(* Logix 5000 Program export KEP; software revision 30.00; part 6 of 15 *)

ADD_ON_INSTRUCTION L_INC   (* revision 1.0 00 Release, vendor Rockwell Automation *)
// Increment (64-bit)
// Revision note:
// Initial Release
// Help:
// This instruction increments the input 64-bit integer, returning its value plus 1.
VAR_IN_OUT
   Inp : LINT; {required}   // Input
   Out : LINT; {required}   // Output = Input + 1
END_VAR
VAR
   Wrk : DINT[2];   // Working pair of 32-bit integers (DINTs)
   Wrk_LoOvflw : BOOL;   // Low-order 32-bit overflow (without minor fault)
   Wrk_HiOvflw : BOOL;   // High-order 32-bit overflow (without minor fault)
END_VAR

ROUTINE Logic   (* ladder *)
// Output the value of the input plus 1
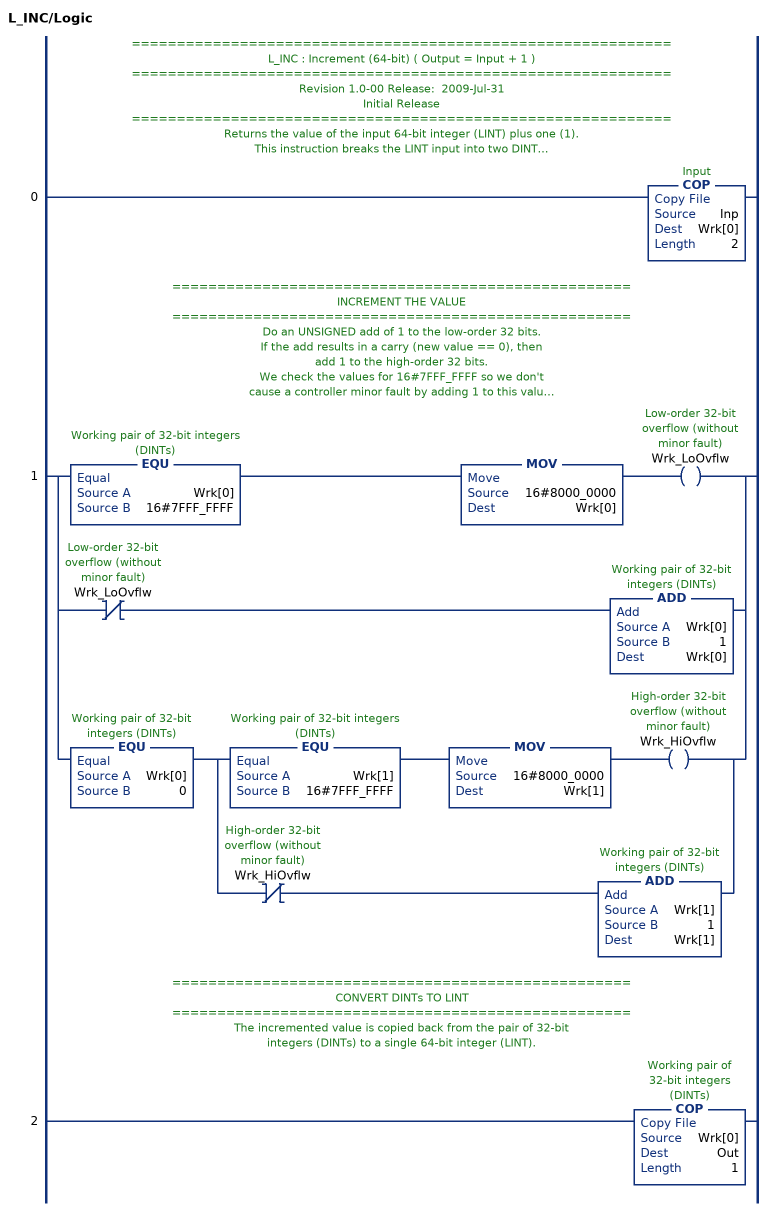
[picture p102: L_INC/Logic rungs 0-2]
   // ============================================================
   // L_INC : Increment (64-bit) ( Output = Input + 1 )
   // ============================================================
   // Revision 1.0-00 Release:  2009-Jul-31
   // Initial Release
   // ============================================================
   // Returns the value of the input 64-bit integer (LINT) plus one (1).
   // This instruction breaks the LINT input into two DINTs
   // (32-bit signed each) to do the math.
   // ===================================================
   // CONVERT LINT TO DINTs
   // ===================================================
   // This COPy takes the input LINT and breaks it into a pair of DINTs.
   0: COP(Inp,Wrk[0],2);
   // ===================================================
   // INCREMENT THE VALUE
   // ===================================================
   // Do an UNSIGNED add of 1 to the low-order 32 bits.
   // If the add results in a carry (new value == 0), then
   // add 1 to the high-order 32 bits.
   // We check the values for 16#7FFF_FFFF so we don't
   // cause a controller minor fault by adding 1 to this value
   // (resulting in a signed overflow to negative).
   1: [EQU(Wrk[0],16#7FFF_FFFF) MOV(16#8000_0000,Wrk[0]) OTE(Wrk_LoOvflw) ,XIO(Wrk_LoOvflw) ADD(Wrk[0],1,Wrk[0]) ,EQU(Wrk[0],0) [EQU(Wrk[1],16#7FFF_FFFF) MOV(16#8000_0000,Wrk[1]) OTE(Wrk_HiOvflw) ,XIO(Wrk_HiOvflw) ADD(Wrk[1],1,Wrk[1]) ] ];
   // ===================================================
   // CONVERT DINTs TO LINT
   // ===================================================
   // The incremented value is copied back from the pair of 32-bit
   // integers (DINTs) to a single 64-bit integer (LINT).
   2: COP(Wrk[0],Out,1);
END_ROUTINE
END_ADD_ON_INSTRUCTION

ADD_ON_INSTRUCTION Ed25519_SIGN   (* revision 1.0 20170916, vendor Kenneth A. Fischer *)
// Generates an Ed25519 Signature.
// Revision note:
// Rev1.0: 20170916 - Initial Release
VAR_IN_OUT
   Temp_C1 : DINT[22]; {required}   // Temp C1 value
   Temp_C2 : DINT[22]; {required}   // Temp C2 value
   Temp_C3 : DINT[22]; {required}   // Temp C3 value
   Temp_C4 : DINT[22]; {required}   // Temp C4 value
   Temp_C5 : DINT[22]; {required}   // Temp C5 value
   Temp_C6 : DINT[22]; {required}   // Temp C6 value
   Temp_C7 : DINT[22]; {required}   // Temp C7 value
   Temp_C8 : DINT[22]; {required}   // Temp C8 value
   Temp_C9 : DINT[22]; {required}   // Temp C9 value
   Temp_C10 : DINT[22]; {required}   // Temp C10 value
   Temp_D1 : DINT[43]; {required}   // Temp D1 Value, w at steps 4/5 and 13/14
   Temp_D2 : DINT[43]; {required}
   Temp_E1 : DINT[32]; {required}   // Temp E1 Value, re
   Temp_E2 : DINT[32]; {required}   // Temp E2 Value, SIG_R between steps 8 and 9, ke for rest
   Temp_E3 : DINT[32]; {required}
   Temp_L : LINT[4]; {required}   // Temp L value
   Temp_S : STRING; {required}   // Temp String
   Temp_P1 : POINT; {required}   // Base Point B
   Temp_P2 : POINT; {required}   // Temp Point for Multiplication
   Temp_P3 : POINT; {required}   // Signature R as Point before encoding
   Temp_P4 : POINT; {required}
   Temp_MSG : LINT[1600]; {required}
   Temp_HASH : LINT[8]; {required}
   Inp_Flags : DINT; {required}
   Inp_PubDH : STRING; {required}
   Inp_Ke : STRING; {required}
   Inp_KsID : LINT; {required}
   Inp_KsPrimeID : LINT; {required}
   Inp_PubKey : STRING; {required}
   Inp_PriKey_scalar : STRING; {required}
   Inp_PriKey_prefix : STRING; {required}
   Out_Counter : LINT; {required}
   Out_Sig_R : STRING; {required}
   Out_Sig_S : STRING; {required}
END_VAR
VAR_OUTPUT
   SEQCTRL_DN : BOOL; {access Read Only}   // Complete
END_VAR
VAR_INPUT
   SEQCTRL_RESET : BOOL;   // Resets Ed25519 Sign if Toggled True
END_VAR
VAR_OUTPUT
   SEQCTRL_STEP : INT; {access Read Only}
   SEQCTRL_SUBSTEP : INT; {access Read Only}
END_VAR
VAR
   SEQCTRL_CMD : DINT;
   SEQCTRL_CMD_TABLE : DINT[70];
   SEQCTRL_DONE : DINT;
   SEQCTRL_NEXT_STEP : INT;
   i : INT;
   TEMP : DINT;
   SHA512_SEQ1 : SHA512_SEQ;
   SEQCTRL_ONS : DINT;
   B512_HtoD : B512_HtoD;
   B256_MODL1 : B256_MODL;
   POINT_MUL : POINT_MUL;
   POINT_ENC : POINT_ENC;
   B256_EtoC : B256_EtoC;
   B256_CtoS : B256_CtoS;
   SHA512_SEQ2 : SHA512_SEQ;
   B256_MODL2 : B256_MODL;
   j : INT;
   B256_NNRED : B256_NNRED;
   B256_EtoL : B256_EtoL;
   B256_StoC : B256_StoC;
   B256_CtoE : B256_CtoE;
   B256_StoSLE : B256_StoSLE;
   Wrk_Out : DINT[2];
   L_INC : L_INC;
END_VAR

ROUTINE Logic   (* ladder *)
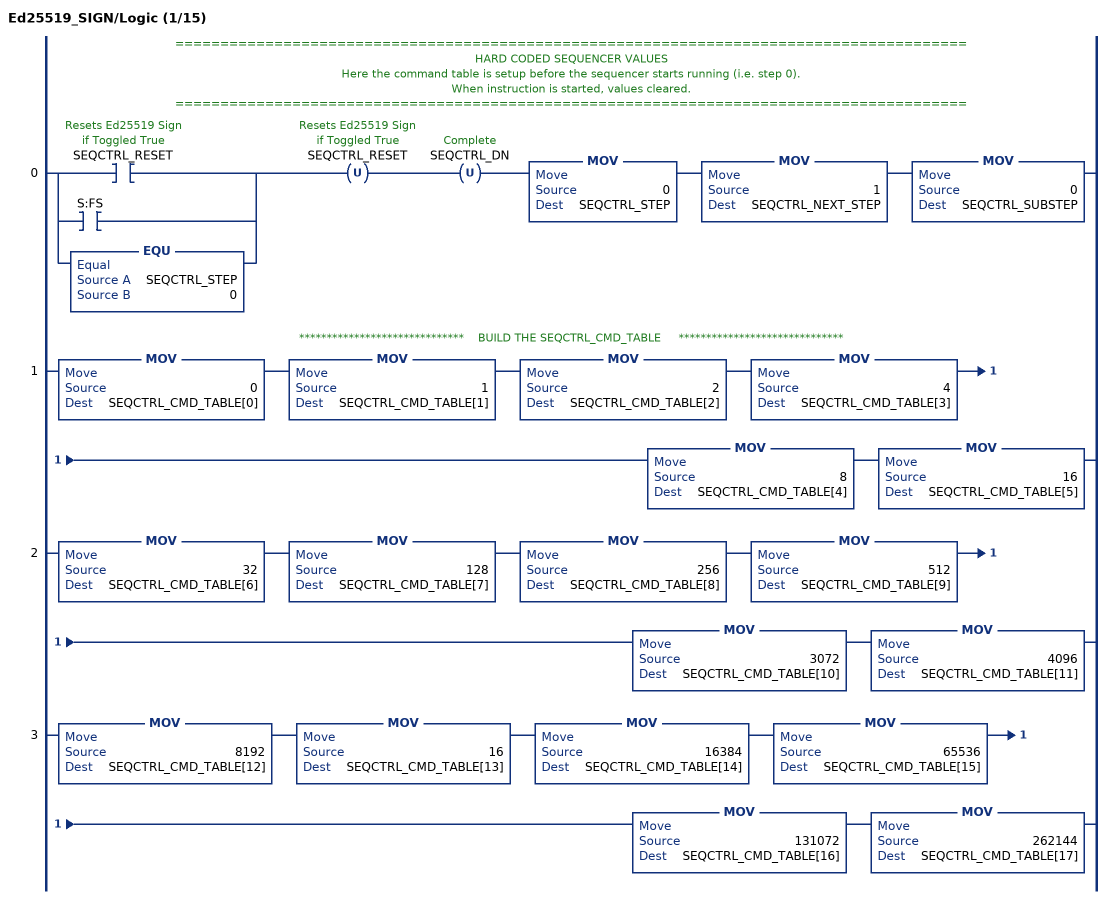
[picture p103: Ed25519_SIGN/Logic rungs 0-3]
   // ========================================================================================
   // HARD CODED SEQUENCER VALUES
   // Here the command table is setup before the sequencer starts running (i.e. step 0).
   // When instruction is started, values cleared.
   // ========================================================================================
   0: [[XIC(SEQCTRL_RESET) ,XIC(S:FS) ] ,EQU(SEQCTRL_STEP,0) ]OTU(SEQCTRL_RESET)OTU(SEQCTRL_DN)MOV(0,SEQCTRL_STEP)MOV(1,SEQCTRL_NEXT_STEP)MOV(0,SEQCTRL_SUBSTEP);
   // ******************************    BUILD THE SEQCTRL_CMD_TABLE     ******************************
   1: MOV(0,SEQCTRL_CMD_TABLE[0])MOV(1,SEQCTRL_CMD_TABLE[1])MOV(2,SEQCTRL_CMD_TABLE[2])MOV(4,SEQCTRL_CMD_TABLE[3])MOV(8,SEQCTRL_CMD_TABLE[4])MOV(16,SEQCTRL_CMD_TABLE[5]);
   2: MOV(32,SEQCTRL_CMD_TABLE[6])MOV(128,SEQCTRL_CMD_TABLE[7])MOV(256,SEQCTRL_CMD_TABLE[8])MOV(512,SEQCTRL_CMD_TABLE[9])MOV(3072,SEQCTRL_CMD_TABLE[10])MOV(4096,SEQCTRL_CMD_TABLE[11]);
   3: MOV(8192,SEQCTRL_CMD_TABLE[12])MOV(16,SEQCTRL_CMD_TABLE[13])MOV(16384,SEQCTRL_CMD_TABLE[14])MOV(65536,SEQCTRL_CMD_TABLE[15])MOV(131072,SEQCTRL_CMD_TABLE[16])MOV(262144,SEQCTRL_CMD_TABLE[17]);
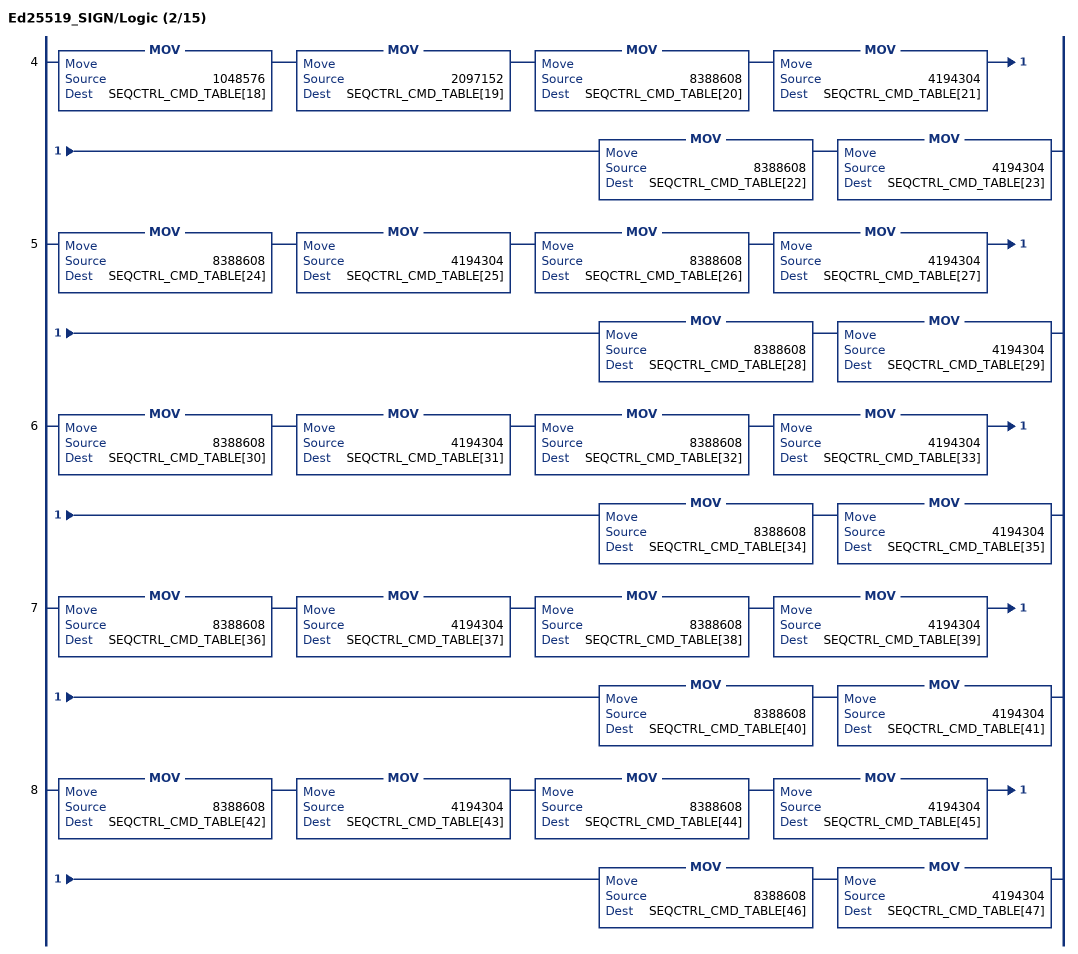
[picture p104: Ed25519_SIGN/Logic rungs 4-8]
   4: MOV(1048576,SEQCTRL_CMD_TABLE[18])MOV(2097152,SEQCTRL_CMD_TABLE[19])MOV(8388608,SEQCTRL_CMD_TABLE[20])MOV(4194304,SEQCTRL_CMD_TABLE[21])MOV(8388608,SEQCTRL_CMD_TABLE[22])MOV(4194304,SEQCTRL_CMD_TABLE[23]);
   5: MOV(8388608,SEQCTRL_CMD_TABLE[24])MOV(4194304,SEQCTRL_CMD_TABLE[25])MOV(8388608,SEQCTRL_CMD_TABLE[26])MOV(4194304,SEQCTRL_CMD_TABLE[27])MOV(8388608,SEQCTRL_CMD_TABLE[28])MOV(4194304,SEQCTRL_CMD_TABLE[29]);
   6: MOV(8388608,SEQCTRL_CMD_TABLE[30])MOV(4194304,SEQCTRL_CMD_TABLE[31])MOV(8388608,SEQCTRL_CMD_TABLE[32])MOV(4194304,SEQCTRL_CMD_TABLE[33])MOV(8388608,SEQCTRL_CMD_TABLE[34])MOV(4194304,SEQCTRL_CMD_TABLE[35]);
   7: MOV(8388608,SEQCTRL_CMD_TABLE[36])MOV(4194304,SEQCTRL_CMD_TABLE[37])MOV(8388608,SEQCTRL_CMD_TABLE[38])MOV(4194304,SEQCTRL_CMD_TABLE[39])MOV(8388608,SEQCTRL_CMD_TABLE[40])MOV(4194304,SEQCTRL_CMD_TABLE[41]);
   8: MOV(8388608,SEQCTRL_CMD_TABLE[42])MOV(4194304,SEQCTRL_CMD_TABLE[43])MOV(8388608,SEQCTRL_CMD_TABLE[44])MOV(4194304,SEQCTRL_CMD_TABLE[45])MOV(8388608,SEQCTRL_CMD_TABLE[46])MOV(4194304,SEQCTRL_CMD_TABLE[47]);
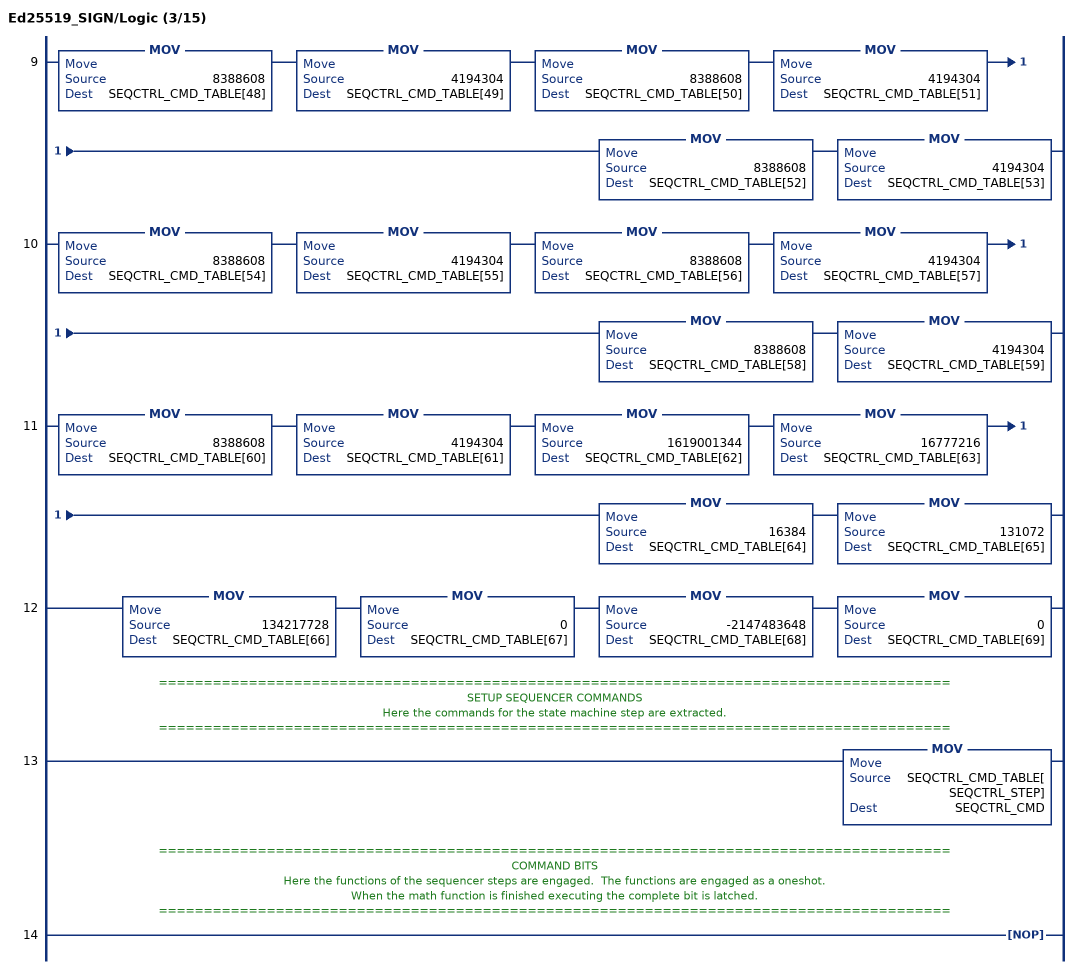
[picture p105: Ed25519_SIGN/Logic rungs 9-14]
   9: MOV(8388608,SEQCTRL_CMD_TABLE[48])MOV(4194304,SEQCTRL_CMD_TABLE[49])MOV(8388608,SEQCTRL_CMD_TABLE[50])MOV(4194304,SEQCTRL_CMD_TABLE[51])MOV(8388608,SEQCTRL_CMD_TABLE[52])MOV(4194304,SEQCTRL_CMD_TABLE[53]);
   10: MOV(8388608,SEQCTRL_CMD_TABLE[54])MOV(4194304,SEQCTRL_CMD_TABLE[55])MOV(8388608,SEQCTRL_CMD_TABLE[56])MOV(4194304,SEQCTRL_CMD_TABLE[57])MOV(8388608,SEQCTRL_CMD_TABLE[58])MOV(4194304,SEQCTRL_CMD_TABLE[59]);
   11: MOV(8388608,SEQCTRL_CMD_TABLE[60])MOV(4194304,SEQCTRL_CMD_TABLE[61])MOV(1619001344,SEQCTRL_CMD_TABLE[62])MOV(16777216,SEQCTRL_CMD_TABLE[63])MOV(16384,SEQCTRL_CMD_TABLE[64])MOV(131072,SEQCTRL_CMD_TABLE[65]);
   12: MOV(134217728,SEQCTRL_CMD_TABLE[66])MOV(0,SEQCTRL_CMD_TABLE[67])MOV(-2147483648,SEQCTRL_CMD_TABLE[68])MOV(0,SEQCTRL_CMD_TABLE[69]);
   // ========================================================================================
   // SETUP SEQUENCER COMMANDS
   // Here the commands for the state machine step are extracted.
   // ========================================================================================
   13: MOV(SEQCTRL_CMD_TABLE[SEQCTRL_STEP],SEQCTRL_CMD);
   // ========================================================================================
   // COMMAND BITS
   // Here the functions of the sequencer steps are engaged.  The functions are engaged as a oneshot.
   // When the math function is finished executing the complete bit is latched.
   // ========================================================================================
   14: NOP();
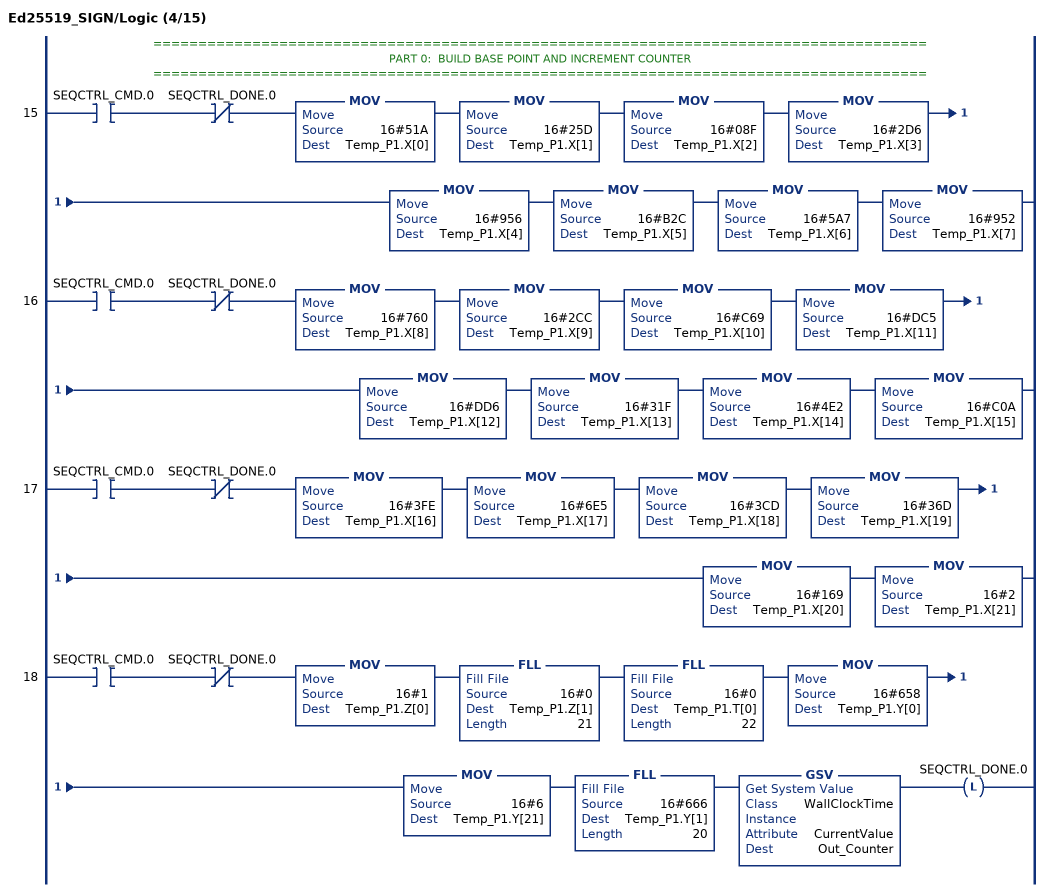
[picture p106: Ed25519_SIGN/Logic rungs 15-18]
   // ======================================================================================
   // PART 0:  BUILD BASE POINT AND INCREMENT COUNTER
   // ======================================================================================
   15: XIC(SEQCTRL_CMD.0)XIO(SEQCTRL_DONE.0)MOV(16#51A,Temp_P1.X[0])MOV(16#25D,Temp_P1.X[1])MOV(16#08F,Temp_P1.X[2])MOV(16#2D6,Temp_P1.X[3])MOV(16#956,Temp_P1.X[4])MOV(16#B2C,Temp_P1.X[5])MOV(16#5A7,Temp_P1.X[6])MOV(16#952,Temp_P1.X[7]);
   16: XIC(SEQCTRL_CMD.0)XIO(SEQCTRL_DONE.0)MOV(16#760,Temp_P1.X[8])MOV(16#2CC,Temp_P1.X[9])MOV(16#C69,Temp_P1.X[10])MOV(16#DC5,Temp_P1.X[11])MOV(16#DD6,Temp_P1.X[12])MOV(16#31F,Temp_P1.X[13])MOV(16#4E2,Temp_P1.X[14])MOV(16#C0A,Temp_P1.X[15]);
   17: XIC(SEQCTRL_CMD.0)XIO(SEQCTRL_DONE.0)MOV(16#3FE,Temp_P1.X[16])MOV(16#6E5,Temp_P1.X[17])MOV(16#3CD,Temp_P1.X[18])MOV(16#36D,Temp_P1.X[19])MOV(16#169,Temp_P1.X[20])MOV(16#2,Temp_P1.X[21]);
   18: XIC(SEQCTRL_CMD.0)XIO(SEQCTRL_DONE.0)MOV(16#1,Temp_P1.Z[0])FLL(16#0,Temp_P1.Z[1],21)FLL(16#0,Temp_P1.T[0],22)MOV(16#658,Temp_P1.Y[0])MOV(16#6,Temp_P1.Y[21])FLL(16#666,Temp_P1.Y[1],20)GSV(WallClockTime,,CurrentValue,Out_Counter)OTL(SEQCTRL_DONE.0);
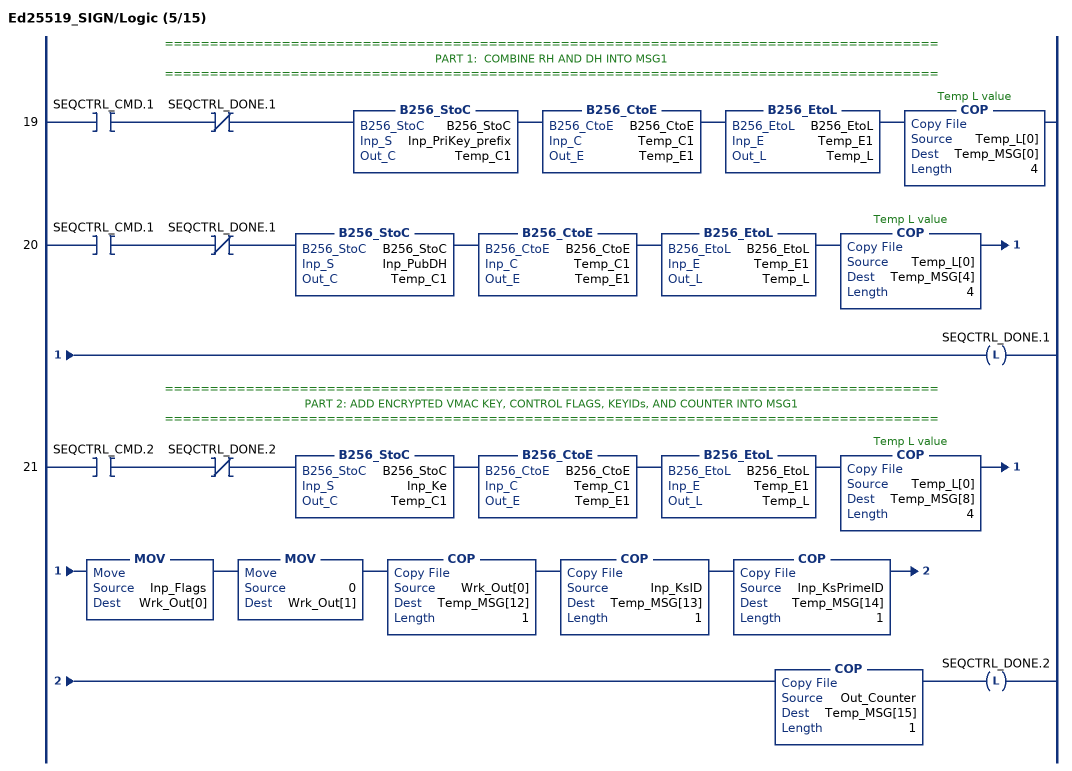
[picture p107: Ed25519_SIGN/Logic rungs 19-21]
   // ======================================================================================
   // PART 1:  COMBINE RH AND DH INTO MSG1
   // ======================================================================================
   19: XIC(SEQCTRL_CMD.1)XIO(SEQCTRL_DONE.1)B256_StoC(B256_StoC,Inp_PriKey_prefix,Temp_C1)B256_CtoE(B256_CtoE,Temp_C1,Temp_E1)B256_EtoL(B256_EtoL,Temp_E1,Temp_L)COP(Temp_L[0],Temp_MSG[0],4);
   20: XIC(SEQCTRL_CMD.1)XIO(SEQCTRL_DONE.1)B256_StoC(B256_StoC,Inp_PubDH,Temp_C1)B256_CtoE(B256_CtoE,Temp_C1,Temp_E1)B256_EtoL(B256_EtoL,Temp_E1,Temp_L)COP(Temp_L[0],Temp_MSG[4],4)OTL(SEQCTRL_DONE.1);
   // ======================================================================================
   // PART 2: ADD ENCRYPTED VMAC KEY, CONTROL FLAGS, KEYIDs, AND COUNTER INTO MSG1
   // ======================================================================================
   21: XIC(SEQCTRL_CMD.2)XIO(SEQCTRL_DONE.2)B256_StoC(B256_StoC,Inp_Ke,Temp_C1)B256_CtoE(B256_CtoE,Temp_C1,Temp_E1)B256_EtoL(B256_EtoL,Temp_E1,Temp_L)COP(Temp_L[0],Temp_MSG[8],4)MOV(Inp_Flags,Wrk_Out[0])MOV(0,Wrk_Out[1])COP(Wrk_Out[0],Temp_MSG[12],1)COP(Inp_KsID,Temp_MSG[13],1)COP(Inp_KsPrimeID,Temp_MSG[14],1)COP(Out_Counter,Temp_MSG[15],1)OTL(SEQCTRL_DONE.2);
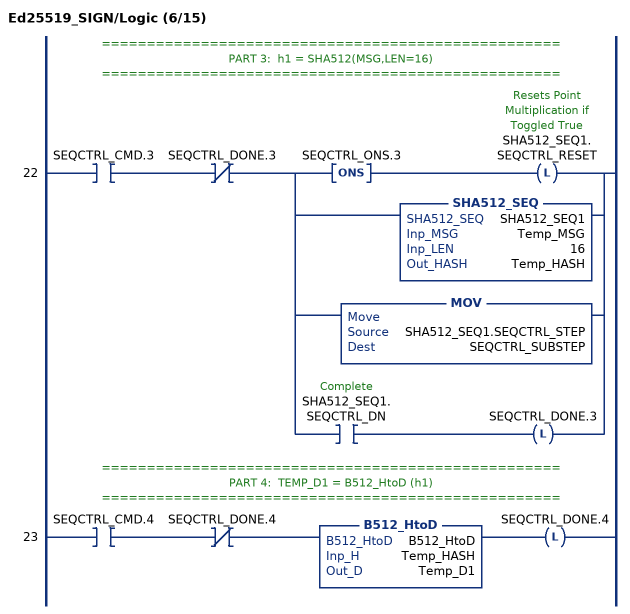
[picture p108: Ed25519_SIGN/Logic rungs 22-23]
   // ===================================================
   // PART 3:  h1 = SHA512(MSG,LEN=16)
   // ===================================================
   22: XIC(SEQCTRL_CMD.3)XIO(SEQCTRL_DONE.3)[ONS(SEQCTRL_ONS.3) OTL(SHA512_SEQ1.SEQCTRL_RESET) ,SHA512_SEQ(SHA512_SEQ1,Temp_MSG,16,Temp_HASH) ,MOV(SHA512_SEQ1.SEQCTRL_STEP,SEQCTRL_SUBSTEP) ,XIC(SHA512_SEQ1.SEQCTRL_DN) OTL(SEQCTRL_DONE.3) ];
   // ===================================================
   // PART 4:  TEMP_D1 = B512_HtoD (h1)
   // ===================================================
   23: XIC(SEQCTRL_CMD.4)XIO(SEQCTRL_DONE.4)B512_HtoD(B512_HtoD,Temp_HASH,Temp_D1)OTL(SEQCTRL_DONE.4);
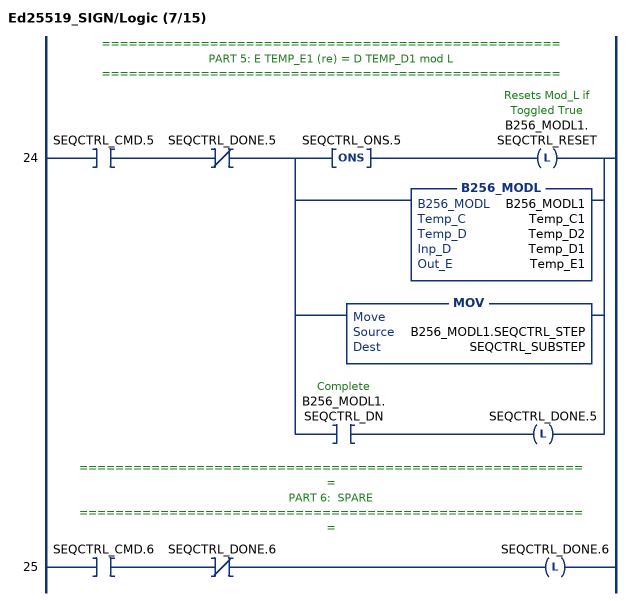
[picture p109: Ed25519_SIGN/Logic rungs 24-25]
   // ===================================================
   // PART 5: E TEMP_E1 (re) = D TEMP_D1 mod L
   // ===================================================
   24: XIC(SEQCTRL_CMD.5)XIO(SEQCTRL_DONE.5)[ONS(SEQCTRL_ONS.5) OTL(B256_MODL1.SEQCTRL_RESET) ,B256_MODL(B256_MODL1,Temp_C1,Temp_D2,Temp_D1,Temp_E1) ,MOV(B256_MODL1.SEQCTRL_STEP,SEQCTRL_SUBSTEP) ,XIC(B256_MODL1.SEQCTRL_DN) OTL(SEQCTRL_DONE.5) ];
   // =========================================================
   // PART 6:  SPARE
   // =========================================================
   25: XIC(SEQCTRL_CMD.6)XIO(SEQCTRL_DONE.6)OTL(SEQCTRL_DONE.6);
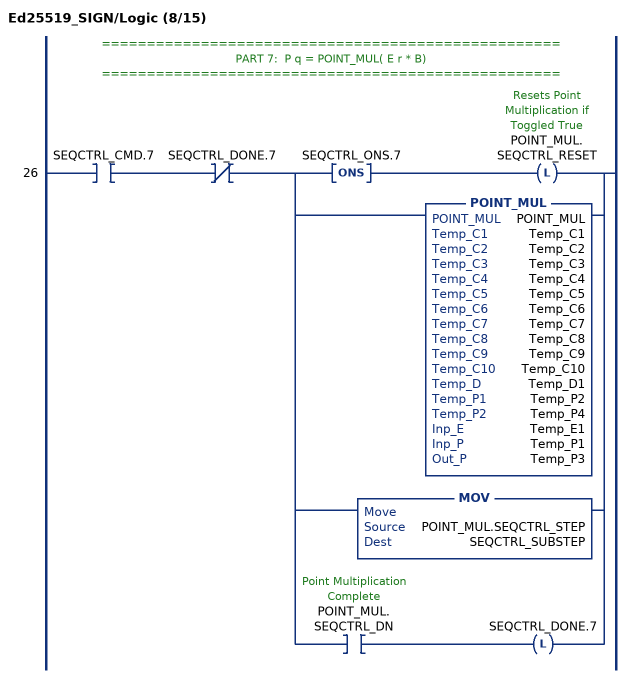
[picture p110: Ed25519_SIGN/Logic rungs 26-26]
   // ===================================================
   // PART 7:  P q = POINT_MUL( E r * B)
   // ===================================================
   26: XIC(SEQCTRL_CMD.7)XIO(SEQCTRL_DONE.7)[ONS(SEQCTRL_ONS.7) OTL(POINT_MUL.SEQCTRL_RESET) ,POINT_MUL(POINT_MUL,Temp_C1,Temp_C2,Temp_C3,Temp_C4,Temp_C5,Temp_C6,Temp_C7,Temp_C8,Temp_C9,Temp_C10,Temp_D1,Temp_P2,Temp_P4,Temp_E1,Temp_P1,Temp_P3) ,MOV(POINT_MUL.SEQCTRL_STEP,SEQCTRL_SUBSTEP) ,XIC(POINT_MUL.SEQCTRL_DN) OTL(SEQCTRL_DONE.7) ];
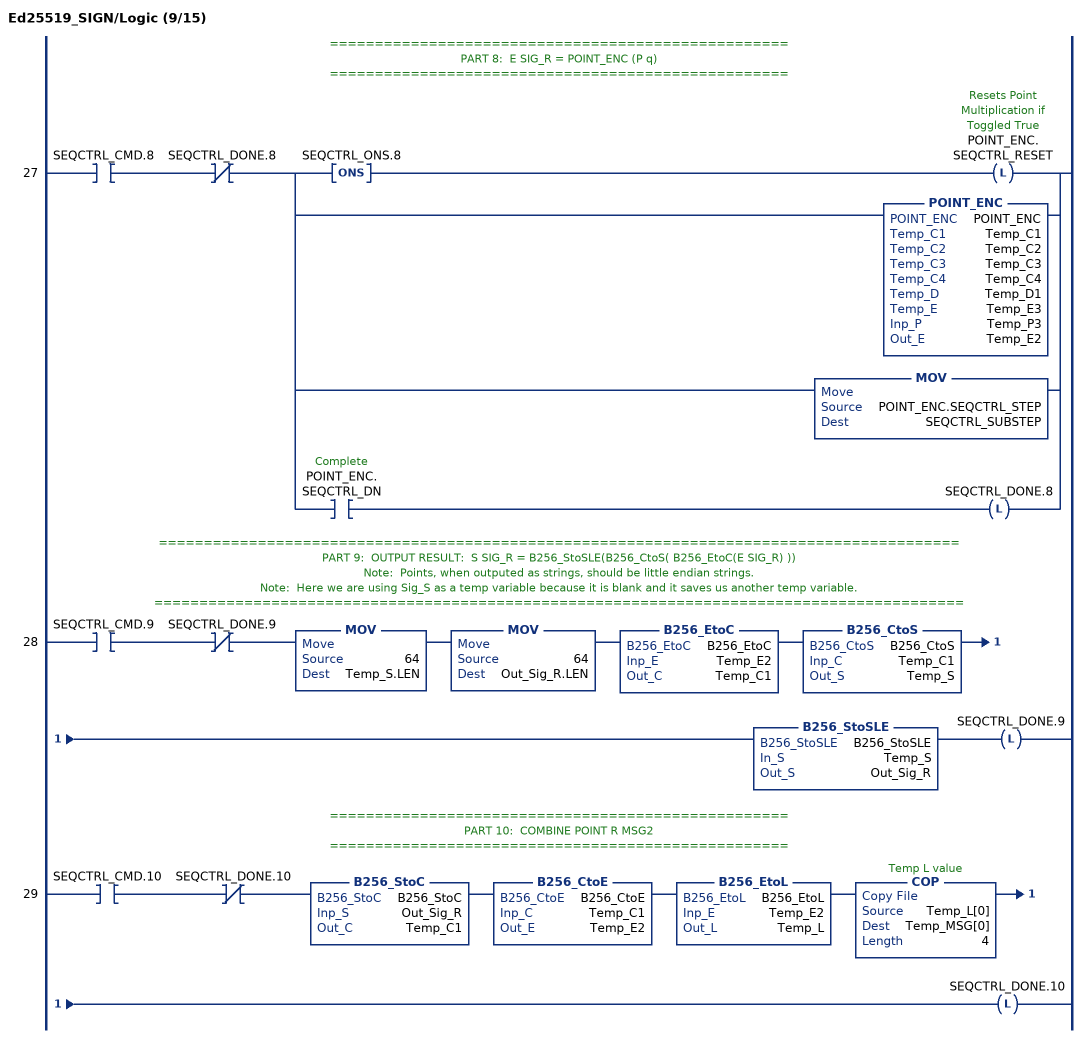
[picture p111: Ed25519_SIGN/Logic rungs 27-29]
   // ===================================================
   // PART 8:  E SIG_R = POINT_ENC (P q)
   // ===================================================
   27: XIC(SEQCTRL_CMD.8)XIO(SEQCTRL_DONE.8)[ONS(SEQCTRL_ONS.8) OTL(POINT_ENC.SEQCTRL_RESET) ,POINT_ENC(POINT_ENC,Temp_C1,Temp_C2,Temp_C3,Temp_C4,Temp_D1,Temp_E3,Temp_P3,Temp_E2) ,MOV(POINT_ENC.SEQCTRL_STEP,SEQCTRL_SUBSTEP) ,XIC(POINT_ENC.SEQCTRL_DN) OTL(SEQCTRL_DONE.8) ];
   // =========================================================================================
   // PART 9:  OUTPUT RESULT:  S SIG_R = B256_StoSLE(B256_CtoS( B256_EtoC(E SIG_R) ))
   // Note:  Points, when outputed as strings, should be little endian strings.
   // Note:  Here we are using Sig_S as a temp variable because it is blank and it saves us another temp variable.
   // ==========================================================================================
   28: XIC(SEQCTRL_CMD.9)XIO(SEQCTRL_DONE.9)MOV(64,Temp_S.LEN)MOV(64,Out_Sig_R.LEN)B256_EtoC(B256_EtoC,Temp_E2,Temp_C1)B256_CtoS(B256_CtoS,Temp_C1,Temp_S)B256_StoSLE(B256_StoSLE,Temp_S,Out_Sig_R)OTL(SEQCTRL_DONE.9);
   // ===================================================
   // PART 10:  COMBINE POINT R MSG2
   // ===================================================
   29: XIC(SEQCTRL_CMD.10)XIO(SEQCTRL_DONE.10)B256_StoC(B256_StoC,Out_Sig_R,Temp_C1)B256_CtoE(B256_CtoE,Temp_C1,Temp_E2)B256_EtoL(B256_EtoL,Temp_E2,Temp_L)COP(Temp_L[0],Temp_MSG[0],4)OTL(SEQCTRL_DONE.10);
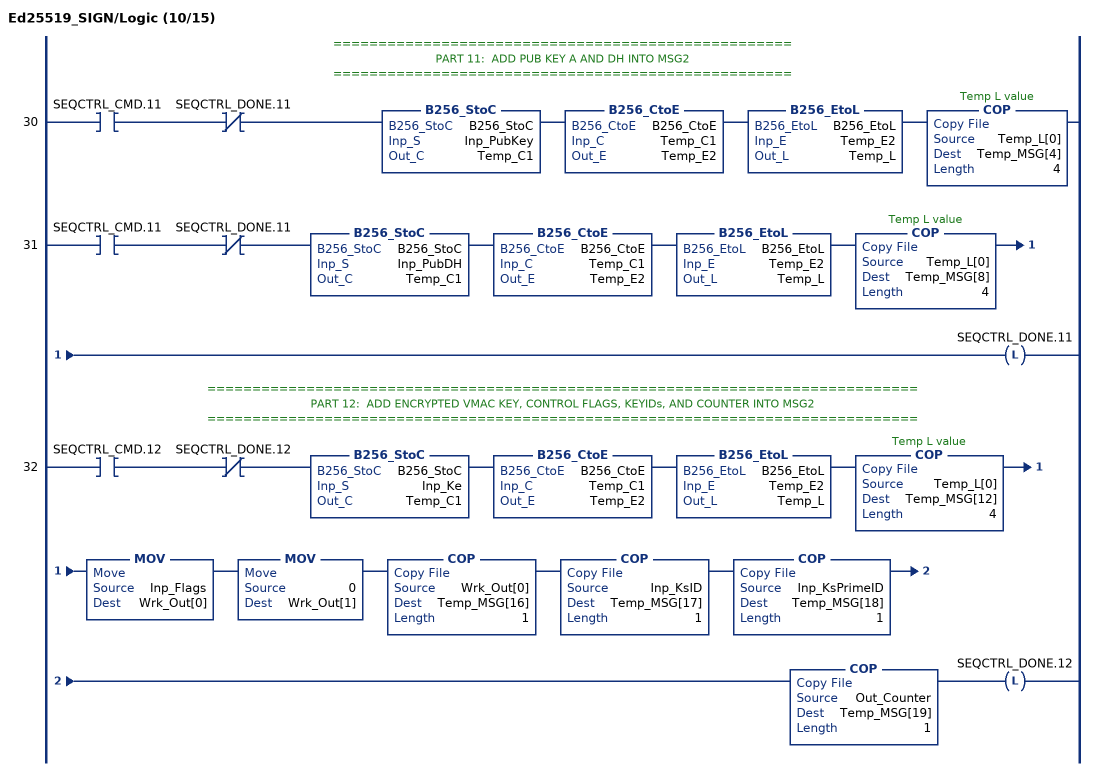
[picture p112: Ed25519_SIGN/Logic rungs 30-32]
   // ===================================================
   // PART 11:  ADD PUB KEY A AND DH INTO MSG2
   // ===================================================
   30: XIC(SEQCTRL_CMD.11)XIO(SEQCTRL_DONE.11)B256_StoC(B256_StoC,Inp_PubKey,Temp_C1)B256_CtoE(B256_CtoE,Temp_C1,Temp_E2)B256_EtoL(B256_EtoL,Temp_E2,Temp_L)COP(Temp_L[0],Temp_MSG[4],4);
   31: XIC(SEQCTRL_CMD.11)XIO(SEQCTRL_DONE.11)B256_StoC(B256_StoC,Inp_PubDH,Temp_C1)B256_CtoE(B256_CtoE,Temp_C1,Temp_E2)B256_EtoL(B256_EtoL,Temp_E2,Temp_L)COP(Temp_L[0],Temp_MSG[8],4)OTL(SEQCTRL_DONE.11);
   // ===============================================================================
   // PART 12:  ADD ENCRYPTED VMAC KEY, CONTROL FLAGS, KEYIDs, AND COUNTER INTO MSG2
   // ===============================================================================
   32: XIC(SEQCTRL_CMD.12)XIO(SEQCTRL_DONE.12)B256_StoC(B256_StoC,Inp_Ke,Temp_C1)B256_CtoE(B256_CtoE,Temp_C1,Temp_E2)B256_EtoL(B256_EtoL,Temp_E2,Temp_L)COP(Temp_L[0],Temp_MSG[12],4)MOV(Inp_Flags,Wrk_Out[0])MOV(0,Wrk_Out[1])COP(Wrk_Out[0],Temp_MSG[16],1)COP(Inp_KsID,Temp_MSG[17],1)COP(Inp_KsPrimeID,Temp_MSG[18],1)COP(Out_Counter,Temp_MSG[19],1)OTL(SEQCTRL_DONE.12);
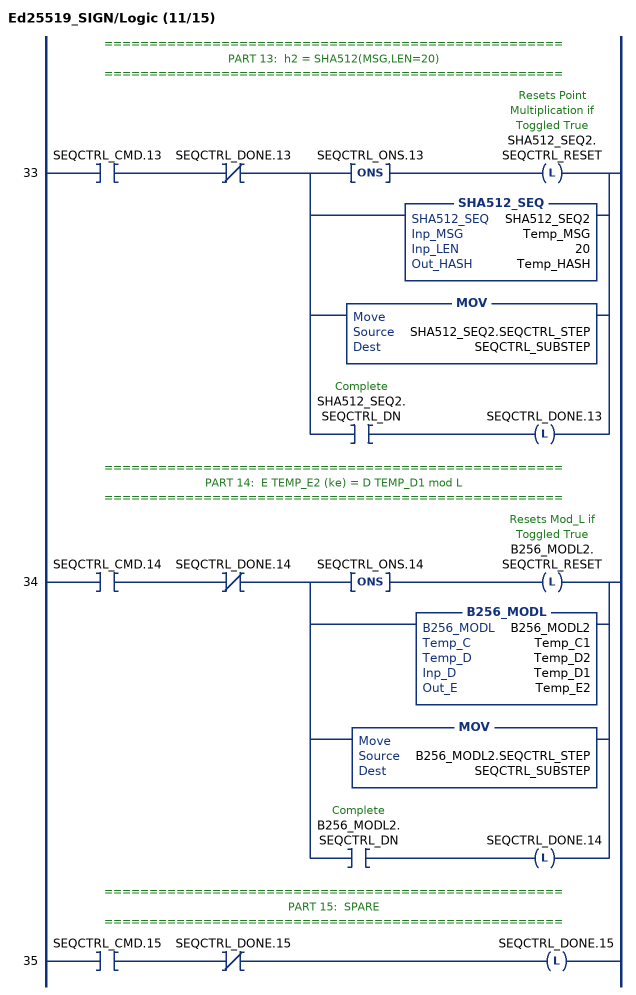
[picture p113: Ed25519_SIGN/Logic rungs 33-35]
   // ===================================================
   // PART 13:  h2 = SHA512(MSG,LEN=20)
   // ===================================================
   33: XIC(SEQCTRL_CMD.13)XIO(SEQCTRL_DONE.13)[ONS(SEQCTRL_ONS.13) OTL(SHA512_SEQ2.SEQCTRL_RESET) ,SHA512_SEQ(SHA512_SEQ2,Temp_MSG,20,Temp_HASH) ,MOV(SHA512_SEQ2.SEQCTRL_STEP,SEQCTRL_SUBSTEP) ,XIC(SHA512_SEQ2.SEQCTRL_DN) OTL(SEQCTRL_DONE.13) ];
   // ===================================================
   // PART 14:  E TEMP_E2 (ke) = D TEMP_D1 mod L
   // ===================================================
   34: XIC(SEQCTRL_CMD.14)XIO(SEQCTRL_DONE.14)[ONS(SEQCTRL_ONS.14) OTL(B256_MODL2.SEQCTRL_RESET) ,B256_MODL(B256_MODL2,Temp_C1,Temp_D2,Temp_D1,Temp_E2) ,MOV(B256_MODL2.SEQCTRL_STEP,SEQCTRL_SUBSTEP) ,XIC(B256_MODL2.SEQCTRL_DN) OTL(SEQCTRL_DONE.14) ];
   // ===================================================
   // PART 15:  SPARE
   // ===================================================
   35: XIC(SEQCTRL_CMD.15)XIO(SEQCTRL_DONE.15)OTL(SEQCTRL_DONE.15);
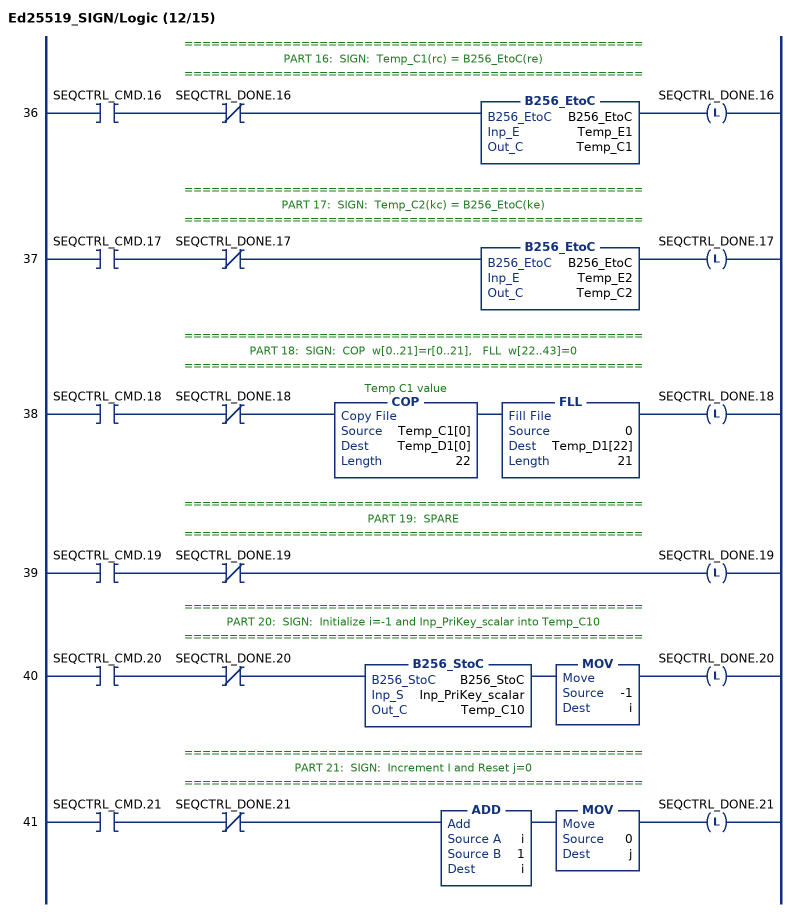
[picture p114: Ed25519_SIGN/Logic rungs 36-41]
   // ===================================================
   // PART 16:  SIGN:  Temp_C1(rc) = B256_EtoC(re)
   // ===================================================
   36: XIC(SEQCTRL_CMD.16)XIO(SEQCTRL_DONE.16)B256_EtoC(B256_EtoC,Temp_E1,Temp_C1)OTL(SEQCTRL_DONE.16);
   // ===================================================
   // PART 17:  SIGN:  Temp_C2(kc) = B256_EtoC(ke)
   // ===================================================
   37: XIC(SEQCTRL_CMD.17)XIO(SEQCTRL_DONE.17)B256_EtoC(B256_EtoC,Temp_E2,Temp_C2)OTL(SEQCTRL_DONE.17);
   // ===================================================
   // PART 18:  SIGN:  COP  w[0..21]=r[0..21],   FLL  w[22..43]=0
   // ===================================================
   38: XIC(SEQCTRL_CMD.18)XIO(SEQCTRL_DONE.18)COP(Temp_C1[0],Temp_D1[0],22)FLL(0,Temp_D1[22],21)OTL(SEQCTRL_DONE.18);
   // ===================================================
   // PART 19:  SPARE
   // ===================================================
   39: XIC(SEQCTRL_CMD.19)XIO(SEQCTRL_DONE.19)OTL(SEQCTRL_DONE.19);
   // ===================================================
   // PART 20:  SIGN:  Initialize i=-1 and Inp_PriKey_scalar into Temp_C10
   // ===================================================
   40: XIC(SEQCTRL_CMD.20)XIO(SEQCTRL_DONE.20)B256_StoC(B256_StoC,Inp_PriKey_scalar,Temp_C10)MOV(-1,i)OTL(SEQCTRL_DONE.20);
   // ===================================================
   // PART 21:  SIGN:  Increment I and Reset j=0
   // ===================================================
   41: XIC(SEQCTRL_CMD.21)XIO(SEQCTRL_DONE.21)ADD(i,1,i)MOV(0,j)OTL(SEQCTRL_DONE.21);
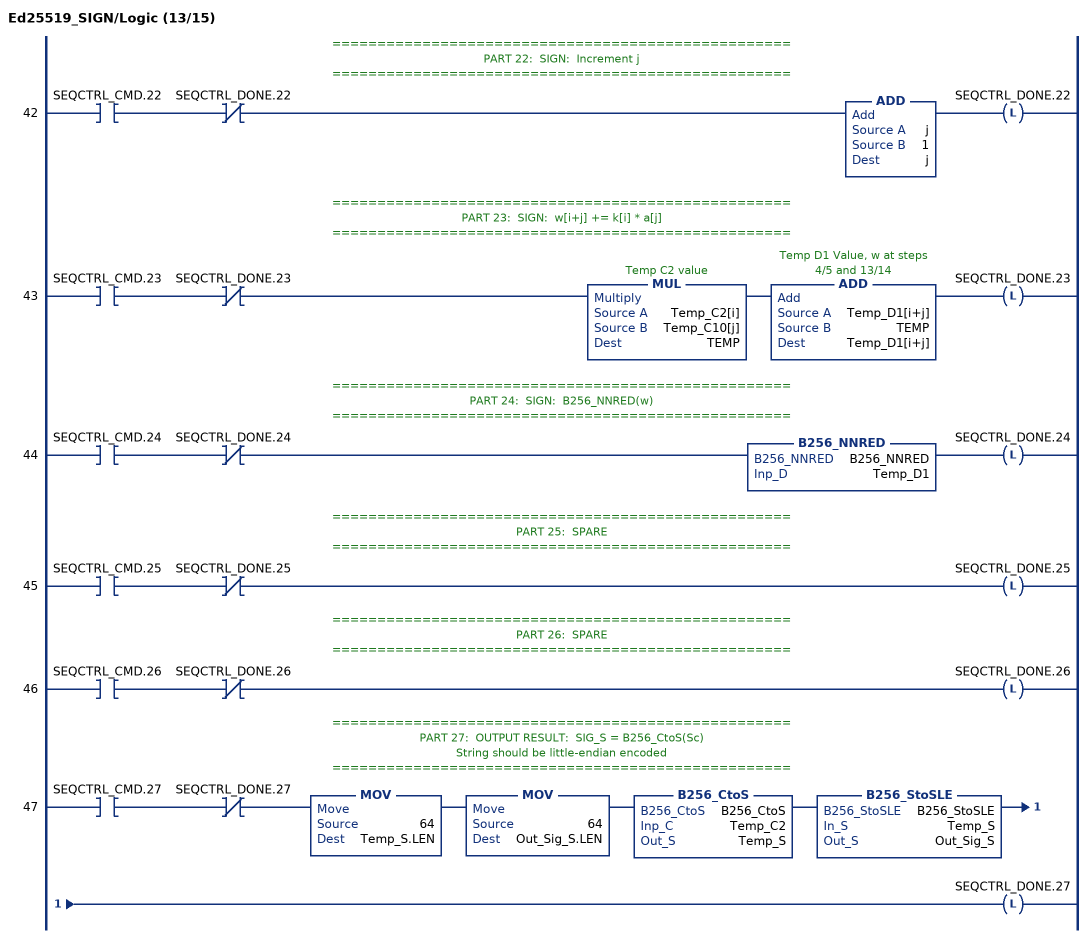
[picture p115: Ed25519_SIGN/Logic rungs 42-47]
   // ===================================================
   // PART 22:  SIGN:  Increment j
   // ===================================================
   42: XIC(SEQCTRL_CMD.22)XIO(SEQCTRL_DONE.22)ADD(j,1,j)OTL(SEQCTRL_DONE.22);
   // ===================================================
   // PART 23:  SIGN:  w[i+j] += k[i] * a[j]
   // ===================================================
   43: XIC(SEQCTRL_CMD.23)XIO(SEQCTRL_DONE.23)MUL(Temp_C2[i],Temp_C10[j],TEMP)ADD(Temp_D1[i+j],TEMP,Temp_D1[i+j])OTL(SEQCTRL_DONE.23);
   // ===================================================
   // PART 24:  SIGN:  B256_NNRED(w)
   // ===================================================
   44: XIC(SEQCTRL_CMD.24)XIO(SEQCTRL_DONE.24)B256_NNRED(B256_NNRED,Temp_D1)OTL(SEQCTRL_DONE.24);
   // ===================================================
   // PART 25:  SPARE
   // ===================================================
   45: XIC(SEQCTRL_CMD.25)XIO(SEQCTRL_DONE.25)OTL(SEQCTRL_DONE.25);
   // ===================================================
   // PART 26:  SPARE
   // ===================================================
   46: XIC(SEQCTRL_CMD.26)XIO(SEQCTRL_DONE.26)OTL(SEQCTRL_DONE.26);
   // ===================================================
   // PART 27:  OUTPUT RESULT:  SIG_S = B256_CtoS(Sc)
   // String should be little-endian encoded
   // ===================================================
   47: XIC(SEQCTRL_CMD.27)XIO(SEQCTRL_DONE.27)MOV(64,Temp_S.LEN)MOV(64,Out_Sig_S.LEN)B256_CtoS(B256_CtoS,Temp_C2,Temp_S)B256_StoSLE(B256_StoSLE,Temp_S,Out_Sig_S)OTL(SEQCTRL_DONE.27);
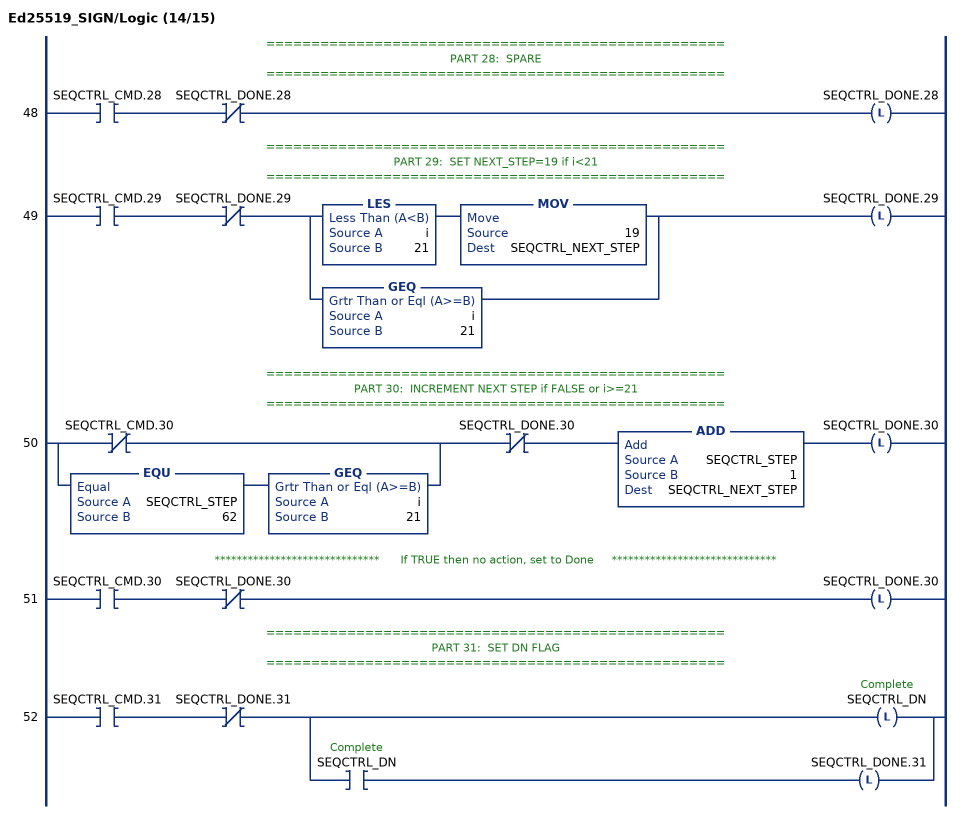
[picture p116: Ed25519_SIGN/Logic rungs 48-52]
   // ===================================================
   // PART 28:  SPARE
   // ===================================================
   48: XIC(SEQCTRL_CMD.28)XIO(SEQCTRL_DONE.28)OTL(SEQCTRL_DONE.28);
   // ===================================================
   // PART 29:  SET NEXT_STEP=19 if i<21
   // ===================================================
   49: XIC(SEQCTRL_CMD.29)XIO(SEQCTRL_DONE.29)[LES(i,21) MOV(19,SEQCTRL_NEXT_STEP) ,GEQ(i,21) ]OTL(SEQCTRL_DONE.29);
   // ===================================================
   // PART 30:  INCREMENT NEXT STEP if FALSE or i>=21
   // ===================================================
   50: [XIO(SEQCTRL_CMD.30) ,EQU(SEQCTRL_STEP,62) GEQ(i,21) ]XIO(SEQCTRL_DONE.30)ADD(SEQCTRL_STEP,1,SEQCTRL_NEXT_STEP)OTL(SEQCTRL_DONE.30);
   // ******************************      If TRUE then no action, set to Done     ******************************
   51: XIC(SEQCTRL_CMD.30)XIO(SEQCTRL_DONE.30)OTL(SEQCTRL_DONE.30);
   // ===================================================
   // PART 31:  SET DN FLAG
   // ===================================================
   52: XIC(SEQCTRL_CMD.31)XIO(SEQCTRL_DONE.31)[OTL(SEQCTRL_DN) ,XIC(SEQCTRL_DN) OTL(SEQCTRL_DONE.31) ];
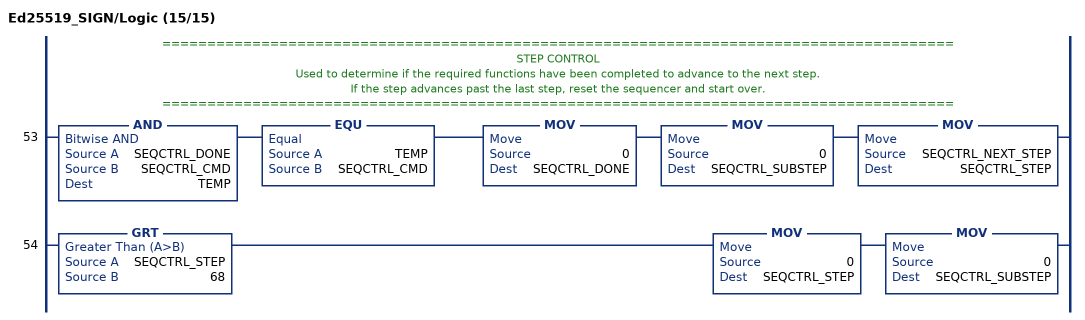
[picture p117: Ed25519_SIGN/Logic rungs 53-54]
   // ========================================================================================
   // STEP CONTROL
   // Used to determine if the required functions have been completed to advance to the next step.
   // If the step advances past the last step, reset the sequencer and start over.
   // ========================================================================================
   53: AND(SEQCTRL_DONE,SEQCTRL_CMD,TEMP)EQU(TEMP,SEQCTRL_CMD)MOV(0,SEQCTRL_DONE)MOV(0,SEQCTRL_SUBSTEP)MOV(SEQCTRL_NEXT_STEP,SEQCTRL_STEP);
   54: GRT(SEQCTRL_STEP,68)MOV(0,SEQCTRL_STEP)MOV(0,SEQCTRL_SUBSTEP);
END_ROUTINE
END_ADD_ON_INSTRUCTION

ADD_ON_INSTRUCTION B256_COMPARE   (* revision 1.0 20170916, vendor Kenneth A. Fischer *)
// Determines if C1<C2, C1=C2, or C1>C2
// Revision note:
// Rev1.0: 20170916 - Initial Release
VAR_IN_OUT
   Inp_C1 : DINT[22]; {required}
   Inp_C2 : DINT[22]; {required}
END_VAR
VAR_OUTPUT
   EQUAL : BOOL; {access Read Only}
   GREATER : BOOL; {access Read Only}
   LESS : BOOL; {access Read Only}
END_VAR
VAR
   C3 : DINT;
   i : DINT;
END_VAR

ROUTINE Logic   (* ladder *)
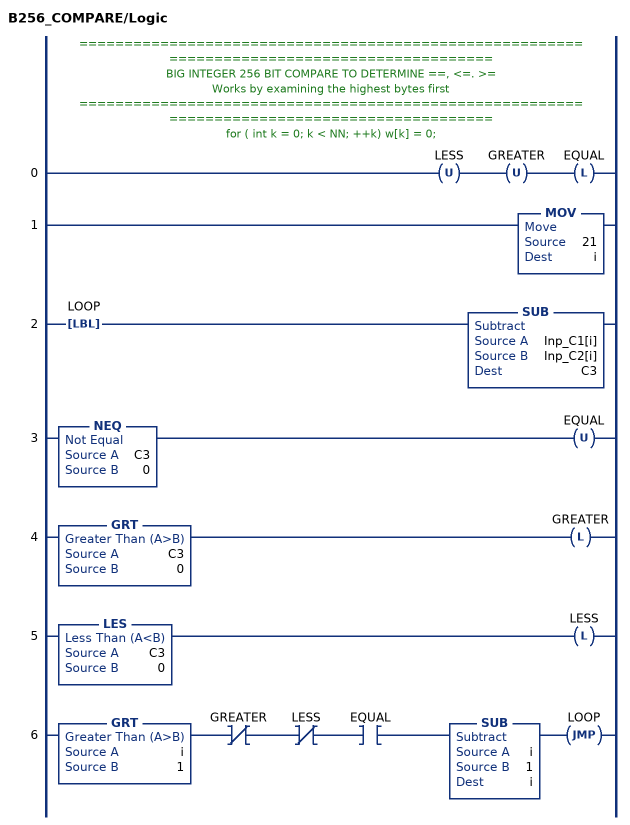
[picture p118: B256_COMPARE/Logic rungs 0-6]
   // ============================================================================================
   // BIG INTEGER 256 BIT COMPARE TO DETERMINE ==, <=. >=
   // Works by examining the highest bytes first
   // ============================================================================================
   // for ( int k = 0; k < NN; ++k) w[k] = 0;
   0: OTU(LESS)OTU(GREATER)OTL(EQUAL);
   1: MOV(21,i);
   2: LBL(LOOP)SUB(Inp_C1[i],Inp_C2[i],C3);
   3: NEQ(C3,0)OTU(EQUAL);
   4: GRT(C3,0)OTL(GREATER);
   5: LES(C3,0)OTL(LESS);
   6: GRT(i,1)XIO(GREATER)XIO(LESS)XIC(EQUAL)SUB(i,1,i)JMP(LOOP);
END_ROUTINE
END_ADD_ON_INSTRUCTION

ADD_ON_INSTRUCTION B256_StoC_LE   (* revision 1.0 20170916, vendor Kenneth A. Fischer *)
// Convert 256-bit value using 64 hex string characters into 256-bit value using 22 12-bit pieces
// Little Endian
// Revision note:
// Rev1.0: 20170916 - Initial Release
VAR_IN_OUT
   Temp_E : DINT[32]; {required}
   Inp_S : STRING; {required}
   Out_C : DINT[22]; {required}
END_VAR
VAR
   byte : DINT[3];
   D_SHL : D_SHL;
   i : INT;
   j : INT;
   k : DINT;
   temp : DINT;
   B256_CtoE : B256_CtoE;
   E : DINT[32];
   B256_EtoC : B256_EtoC;
END_VAR

ROUTINE Logic   (* ladder *)
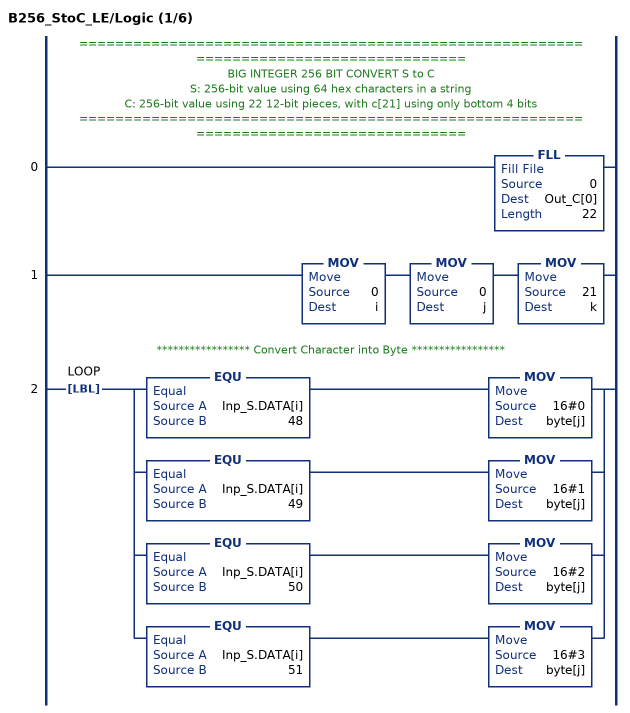
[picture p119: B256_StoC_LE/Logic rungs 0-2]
   // ======================================================================================
   // BIG INTEGER 256 BIT CONVERT S to C
   // S: 256-bit value using 64 hex characters in a string
   // C: 256-bit value using 22 12-bit pieces, with c[21] using only bottom 4 bits
   // ======================================================================================
   0: FLL(0,Out_C[0],22);
   1: MOV(0,i)MOV(0,j)MOV(21,k);
   // ***************** Convert Character into Byte *****************
   2: LBL(LOOP)[EQU(Inp_S.DATA[i],48) MOV(16#0,byte[j]) ,EQU(Inp_S.DATA[i],49) MOV(16#1,byte[j]) ,EQU(Inp_S.DATA[i],50) MOV(16#2,byte[j]) ,EQU(Inp_S.DATA[i],51) MOV(16#3,byte[j]) ];
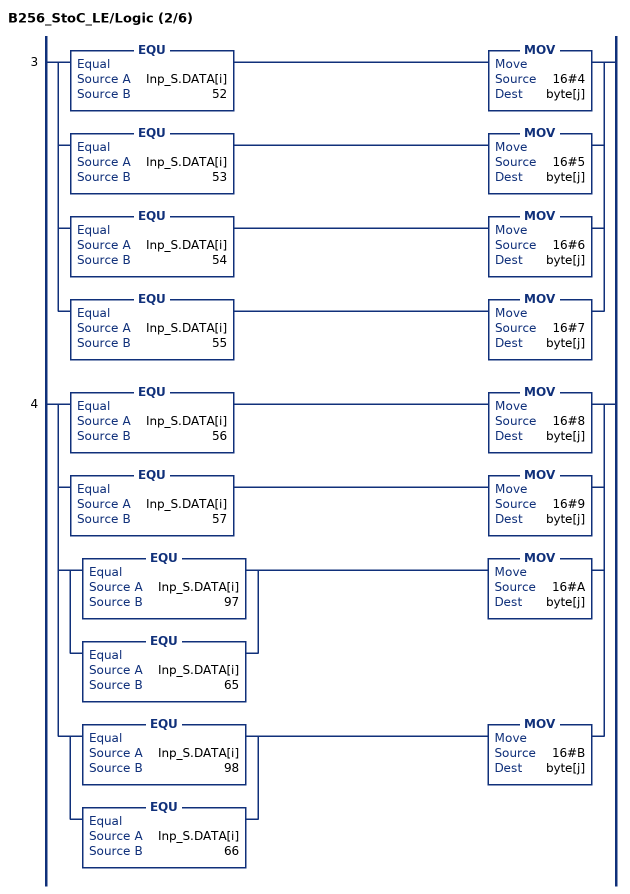
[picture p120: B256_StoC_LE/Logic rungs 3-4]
   3: [EQU(Inp_S.DATA[i],52) MOV(16#4,byte[j]) ,EQU(Inp_S.DATA[i],53) MOV(16#5,byte[j]) ,EQU(Inp_S.DATA[i],54) MOV(16#6,byte[j]) ,EQU(Inp_S.DATA[i],55) MOV(16#7,byte[j]) ];
   4: [EQU(Inp_S.DATA[i],56) MOV(16#8,byte[j]) ,EQU(Inp_S.DATA[i],57) MOV(16#9,byte[j]) ,[EQU(Inp_S.DATA[i],97) ,EQU(Inp_S.DATA[i],65) ] MOV(16#A,byte[j]) ,[EQU(Inp_S.DATA[i],98) ,EQU(Inp_S.DATA[i],66) ] MOV(16#B,byte[j]) ];
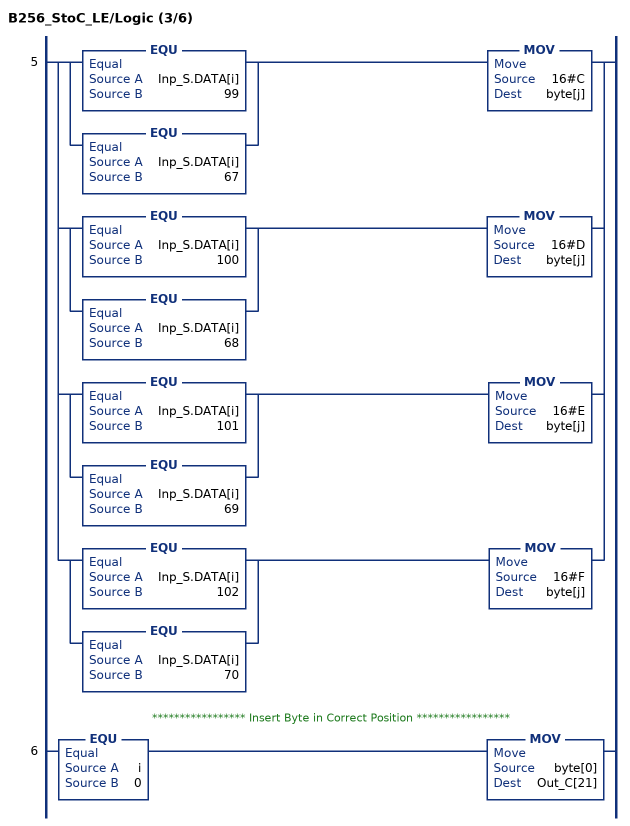
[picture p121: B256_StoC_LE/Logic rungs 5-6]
   5: [[EQU(Inp_S.DATA[i],99) ,EQU(Inp_S.DATA[i],67) ] MOV(16#C,byte[j]) ,[EQU(Inp_S.DATA[i],100) ,EQU(Inp_S.DATA[i],68) ] MOV(16#D,byte[j]) ,[EQU(Inp_S.DATA[i],101) ,EQU(Inp_S.DATA[i],69) ] MOV(16#E,byte[j]) ,[EQU(Inp_S.DATA[i],102) ,EQU(Inp_S.DATA[i],70) ] MOV(16#F,byte[j]) ];
   // ***************** Insert Byte in Correct Position *****************
   6: EQU(i,0)MOV(byte[0],Out_C[21]);
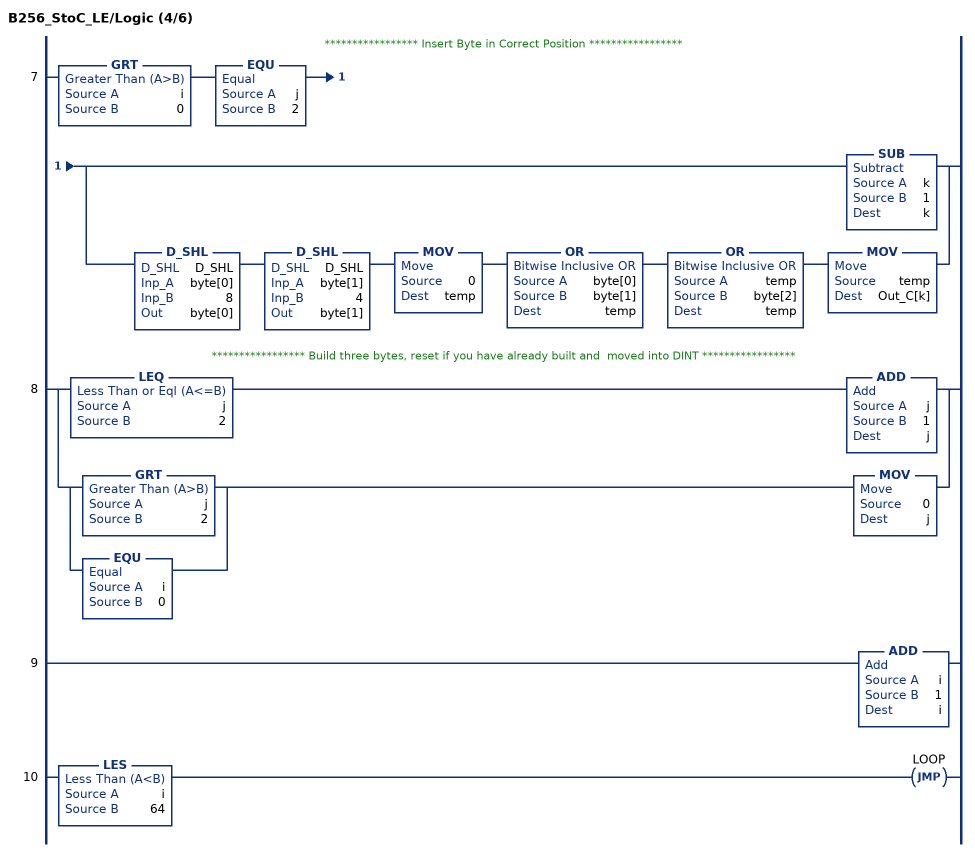
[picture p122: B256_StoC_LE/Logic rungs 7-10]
   // ***************** Insert Byte in Correct Position *****************
   7: GRT(i,0)EQU(j,2)[SUB(k,1,k) ,D_SHL(D_SHL,byte[0],8,byte[0]) D_SHL(D_SHL,byte[1],4,byte[1]) MOV(0,temp) OR(byte[0],byte[1],temp) OR(temp,byte[2],temp) MOV(temp,Out_C[k]) ];
   // ***************** Build three bytes, reset if you have already built and  moved into DINT *****************
   8: [LEQ(j,2) ADD(j,1,j) ,[GRT(j,2) ,EQU(i,0) ] MOV(0,j) ];
   9: ADD(i,1,i);
   10: LES(i,64)JMP(LOOP);
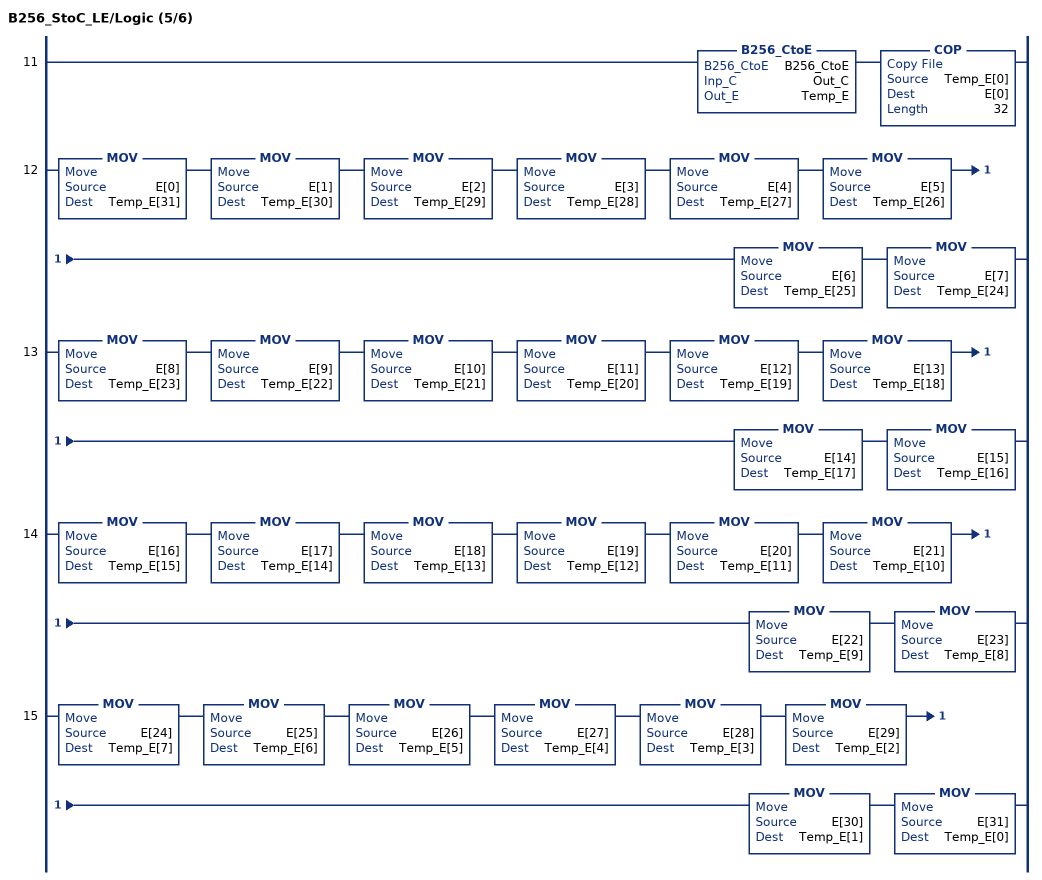
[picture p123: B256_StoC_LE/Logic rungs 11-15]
   11: B256_CtoE(B256_CtoE,Out_C,Temp_E)COP(Temp_E[0],E[0],32);
   12: MOV(E[0],Temp_E[31])MOV(E[1],Temp_E[30])MOV(E[2],Temp_E[29])MOV(E[3],Temp_E[28])MOV(E[4],Temp_E[27])MOV(E[5],Temp_E[26])MOV(E[6],Temp_E[25])MOV(E[7],Temp_E[24]);
   13: MOV(E[8],Temp_E[23])MOV(E[9],Temp_E[22])MOV(E[10],Temp_E[21])MOV(E[11],Temp_E[20])MOV(E[12],Temp_E[19])MOV(E[13],Temp_E[18])MOV(E[14],Temp_E[17])MOV(E[15],Temp_E[16]);
   14: MOV(E[16],Temp_E[15])MOV(E[17],Temp_E[14])MOV(E[18],Temp_E[13])MOV(E[19],Temp_E[12])MOV(E[20],Temp_E[11])MOV(E[21],Temp_E[10])MOV(E[22],Temp_E[9])MOV(E[23],Temp_E[8]);
   15: MOV(E[24],Temp_E[7])MOV(E[25],Temp_E[6])MOV(E[26],Temp_E[5])MOV(E[27],Temp_E[4])MOV(E[28],Temp_E[3])MOV(E[29],Temp_E[2])MOV(E[30],Temp_E[1])MOV(E[31],Temp_E[0]);
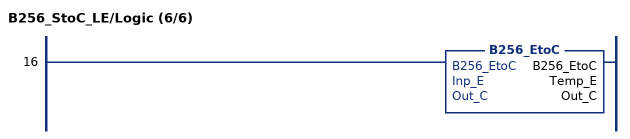
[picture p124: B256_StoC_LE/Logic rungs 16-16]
   16: B256_EtoC(B256_EtoC,Temp_E,Out_C);
END_ROUTINE
END_ADD_ON_INSTRUCTION
